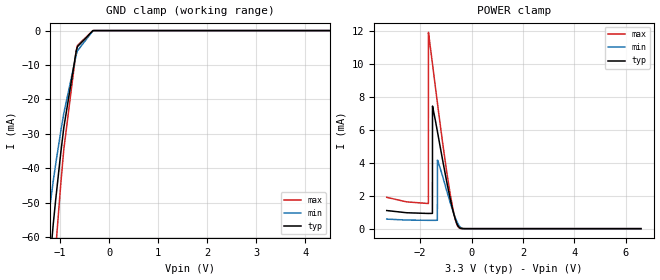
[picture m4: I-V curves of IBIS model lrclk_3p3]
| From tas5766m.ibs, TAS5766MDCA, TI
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|   lrclk_3p3 Model
[Model]   lrclk_3p3
Model_type   Input
Vinl = 0.8
Vinh = 2
|   typ   min   max
|   (nom PVT)   (fast PVT)   (slow PVT)
C_comp   6.403e-12   5.917e-12   6.668e-12
| Where nom  PVT is Nominal Process, 3.3V, 27C
|   Fast PVT is Strong Process,  3.6V, -40C
|   Slow PVT is Weak Process,   3V, 125C
[Voltage Range]   3.3   3   3.6
|Junction Temperature
[Temperature Range]   27   125   -40
[Power Clamp Reference]   3.3   3   3.6
[GND Clamp Reference]   0   0   0
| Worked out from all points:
|   POWER clamp passes 1 mA (typ) near -0.71 V on its own axis
[GND Clamp]
|   Voltage   I(typ)   I(min)   I(max)
-3.3V     -1.542A    -1.263A    -1.822A
-1.373V   -93.75mA   -69.09mA   -125.9mA
-1.14V    -56.29mA   -43.7mA    -73.49mA
-1.086V   -48.56mA   -38.37mA   -62.69mA
-986.7mV  -35.57mA   -29.3mA    -44.65mA
-924mV    -28.14mA   -24.02mA   -34.45mA
-672mV    -6.037mA   -7.11mA    -5.9mA
-646.8mV  -4.683mA   -5.888mA   -4.309mA
-330mV    -4.074uA   -38.34uA   -407.4nA
6.6V      0A         0A         0A
[POWER Clamp]
|   Voltage   I(typ)   I(min)   I(max)
-3.3V     1.099mA    579.3uA    1.9mA
-1.68V    922uA      505.5uA    1.525mA
-1.676V   922uA      505.5uA    11.9mA
-1.521V   925.9uA    504.4uA    10.02mA
-1.518V   7.435mA    504.4uA    9.976mA
-1.329V   5.906mA    512.3uA    7.65mA
-1.326V   5.881mA    4.158mA    7.613mA
-973.5mV  2.914mA    2.346mA    3.541mA
-816mV    1.717mA    1.515mA    1.983mA
-628.8mV  564.9uA    650.4uA    545.9uA
-483mV    80.45uA    179.4uA    42.25uA
6.6V      0A         0A         0A
